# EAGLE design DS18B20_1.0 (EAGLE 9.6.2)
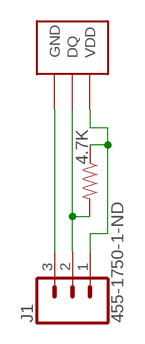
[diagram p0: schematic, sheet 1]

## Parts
4.7K  RESISTORAXIAL-0.3  [AXIAL-0.3]
J1  455-1750-1-ND  CONN_03  [1X03]
X1  DS18B20-TO92  [TO92]

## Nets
N$6: 4.7K.P$2 J1.2 X1.2(DQ)
N$7: 4.7K.P$1 J1.1 X1.3(VDD)
N$8: J1.3 X1.1(GND)

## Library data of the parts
4.7K = SparkFun-Resistors:RESISTOR: Generic Resistor Package
J1 = SparkFun-Connectors:CONN_03: Multi connection point. Often used as Generic Header-pin footprint for 0.1 inch spaced/style header connections On any of the 0.1 inch spaced packages, you can populate with these: Break Away Headers - Straight (PRT-00116) Break Away Male Headers - Right Angle (PRT-00553) Female Headers (PRT-00115)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; PROD_ID: XXX-00000
X1 = kanflo:DS18B20: Dallas DS18B20 1-wire temperature sensor.

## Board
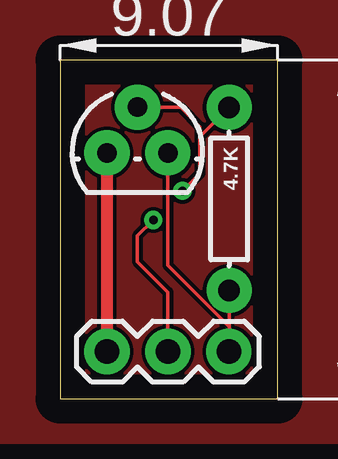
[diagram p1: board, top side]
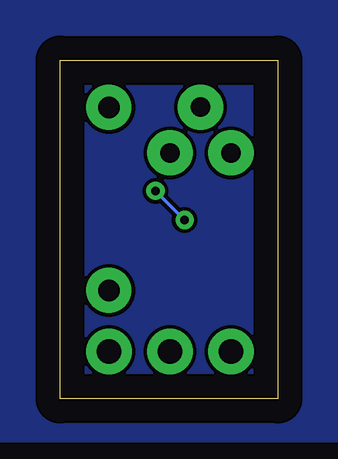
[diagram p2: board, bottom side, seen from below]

Size 9.08 x 14.12 mm. Coordinates in mm from the lower left corner, seen from the top.
Outline: 0,0 9.08,0 9.08,14.12 0,14.11 0,0
Copper layers (1*16): Top 0.035mm / dielectric 1.5mm / Bottom 0.035mm
Design rules "default": minimum track width 6mil, minimum drill 0.35mm, track to track 6mil, track to pad 6mil, pad to pad 6mil, via to via 6mil, smd to smd 6mil, copper to edge 40mil, drill to drill 6mil, minimum pad ring 10mil, minimum via ring 8mil, stop-mask expansion 4mil, vias tented up to drill 0mil, thermal gap 10mil

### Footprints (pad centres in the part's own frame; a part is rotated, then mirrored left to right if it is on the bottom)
AXIAL-0.3 = drill 0.9 pad 1.88: P$1 -3.81,0; P$2 3.81,0
1X03 = drill 1.016 pad 1.88: 1 0,0; 2 2.54,0; 3 5.08,0
TO92 = drill 0.813 pad 1.88: 1 -1.27,1.27; 2 0,3.175; 3 1.27,1.27

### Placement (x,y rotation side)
4.7K  7.05,8.33 90 top
J1  7.04,1.97 180 top
X1  3.23,8.98 0 top

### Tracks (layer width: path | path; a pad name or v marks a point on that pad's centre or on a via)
GND_ACTUATOR
  pour Top: -4.15,19.44 -4.15,-1.81 15.91,-1.81 15.91,19.44
  pour Bottom: -5.76,19.96 -5.76,-1.75 16.74,-1.75 16.74,19.96
N$6  (via drill 0.35)
  Top 0.152: X1.2 3.24,12.14 5.03,12.14 5.83,11.34 5.83,10.92 | J1.2 4.5,4.44 3.23,5.72 3.23,6.79 v3.89,7.45 | 5.83,10.92 5.83,9.38 v5.11,8.66 | 4.7K.P$2 5.83,10.92
  Bottom 0.152: v5.11,8.66 v3.89,7.45
N$7
  Top 0.152: 7.05,3 7.05,1.98 J1.1 | X1.3 4.5,5.56 7.05,3 | 7.05,3 4.7K.P$1
N$8
  Top 0.152: J1.3
  Top 0.508: X1.1 J1.3

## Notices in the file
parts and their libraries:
SparkFun-Resistors: Licensing: Creative Commons ShareAlike 4.0 International - https://creativecommons.org/licenses/by-sa/4.0
